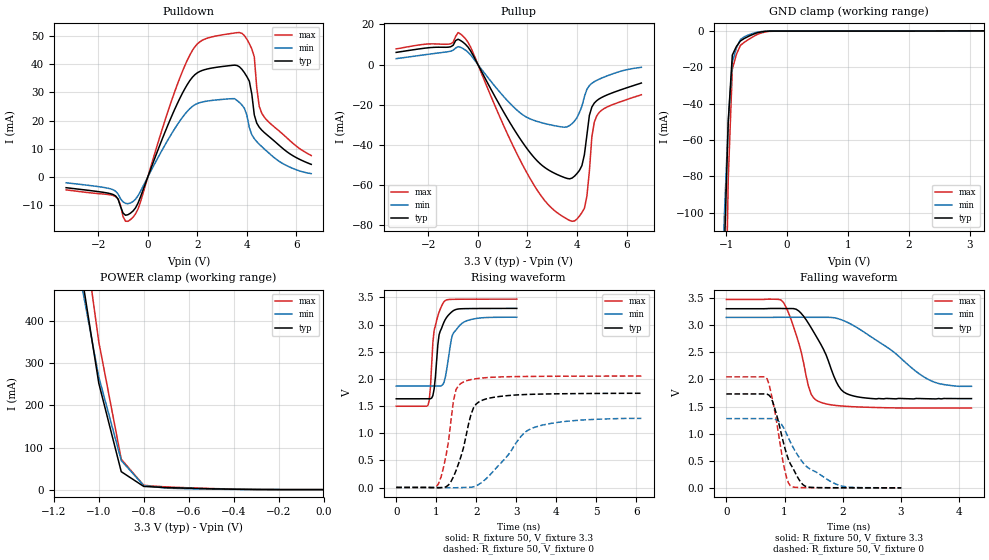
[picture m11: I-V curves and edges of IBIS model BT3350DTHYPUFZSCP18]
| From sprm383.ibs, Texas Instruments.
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|   Model Cell BT3350DTHYPUFZSCP18
[Model]   BT3350DTHYPUFZSCP18
Model_type   I/O
Polarity   Non-Inverting
Enable   Active-Low
Vinl =  0.8V
Vinh =  2V
Cref =  15.0000pF
Rref =  100.0000M
Vref =  0V
Vmeas =  1.65
C_comp   1.486782p   1.450653p   1.527115p
[Model Spec]
Vinl   0.8V   0.8V   0.8V
Vinh   2V   2V   2V
[Temperature Range]   25   105   0
[Voltage Range]   3.3   3.14   3.47
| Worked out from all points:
|   slope of the pulldown table from 0 to 0.495 V, typ, clamps not added: 43 ohm
|   slope of the pullup table from 0 to 0.495 V, typ, clamps not added: 42.8 ohm
|   GND clamp passes 1 mA (typ) near -0.48 V on its own axis
|   POWER clamp passes 1 mA (typ) near -0.41 V on its own axis
|   rising waveform, R_fixture 50, V_fixture 3.3: 20-80 % time 180ps typ, 223ps min, 150ps max; typ from 1.64 V to 3.3 V
|   rising waveform, R_fixture 50, V_fixture 0: 20-80 % time 378ps typ, 854ps min, 250ps max; typ from 0.003 V to 1.74 V
|   falling waveform, R_fixture 50, V_fixture 3.3: 20-80 % time 434ps typ, 942ps min, 290ps max; typ from 3.3 V to 1.65 V
|   falling waveform, R_fixture 50, V_fixture 0: 20-80 % time 298ps typ, 570ps min, 197ps max; typ from 1.73 V to 0.004 V
[POWER_clamp]
|   voltage   I(typ)   I(min)   I(max)
-3.3V     9.961A     8.611A     10.94A
-1.067V   478.9mA    459.3mA    610.8mA
-1.033V   365.9mA    363.6mA    481.1mA
-1V       253mA      268mA      351.4mA
-900mV    42.61mA    69.09mA    72.29mA
-800mV    7.588mA    9.637mA    10.15mA
-700mV    4.837mA    3.413mA    6.304mA
-600mV    3.264mA    2.054mA    4.281mA
-300mV    294.4uA    124uA      421.6uA
-11.55fV  111.8nA    122.7nA    532.3nA
[Pulldown]
|   voltage   I(typ)   I(min)   I(max)
-3.3V     -3.799mA   -2.054mA   -4.568mA
-1.3V     -6.728mA   -5.045mA   -6.952mA
-700mV    -12.84mA   -9.218mA   -15.12mA
-400mV    -9.372mA   -6.707mA   -11.45mA
900mV     20.28mA    14.47mA    25.55mA
1.8V      35.39mA    25.05mA    44.9mA
3.6V      39.59mA    27.18mA    51.23mA
4.1V      33.99mA    17.52mA    47.31mA
4.3V      22.03mA    13.6mA     42.63mA
4.4V      19.11mA    12.56mA    31.7mA
4.6V      16.65mA    10.8mA     22.67mA
6.6V      4.483mA    1.197mA    7.628mA
[Pullup]
|   voltage   I(typ)   I(min)   I(max)
-3.3V     6.066mA    2.957mA    7.802mA
-600mV    11.14mA    7.958mA    14.14mA
1.3V      -29.12mA   -19.42mA   -37.44mA
2.2V      -45.34mA   -27.53mA   -58.77mA
2.9V      -52.9mA    -29.98mA   -70.61mA
3.8V      -56.58mA   -29.42mA   -78.12mA
4.3V      -44.86mA   -15.96mA   -71.64mA
4.4V      -35.19mA   -12.35mA   -65.67mA
4.5V      -25.37mA   -10.47mA   -53.29mA
4.6V      -21.19mA   -9.34mA    -36.14mA
4.8V      -17.96mA   -7.847mA   -25.51mA
6.6V      -9.2mA     -1.379mA   -15.05mA
[GND_clamp]
|   voltage   I(typ)   I(min)   I(max)
-3.3V     -13.48A    -11.6A     -14.64A
-1.1V     -237.6mA   -179.7mA   -391.1mA
-1.033V   -124.3mA   -104mA     -204.7mA
-966.7mV  -49.58mA   -49.82mA   -81.35mA
-900mV    -13.35mA   -17.24mA   -21.09mA
-833.3mV  -8.63mA    -9.469mA   -12.94mA
-766.7mV  -5.563mA   -4.788mA   -7.981mA
-700mV    -4.145mA   -3.193mA   -6.208mA
-500mV    -1.148mA   -798uA     -2.146mA
-300mV    -166.1uA   -102.4uA   -290.3uA
3.233V    -8.734uA   9.395uA    -38.37uA
[Ramp]
| variable   typ   min   max
dV/dt_f   1.026406/0.448073n   0.8129736/1.011668n   1.202557/0.2908703n
dV/dt_r   1.048978/0.378546n   0.79136/0.9065475n   1.235918/0.2476382n
R_load = 50
[Rising Waveform]
R_fixture = 50
V_fixture = 3.3
V_fixture_min = 3.14
V_fixture_max = 3.47
|   time   V(typ)   V(min)   V(max)
0s        1.635V     1.869V     1.498V
796ps     1.636V     1.87V      1.519V
856ps     1.636V     1.87V      1.854V
916ps     1.694V     1.87V      2.674V
948ps     1.818V     1.87V      2.898V
1.072ns   2.817V     1.87V      3.232V
1.224ns   3.092V     2.02V      3.443V
1.408ns   3.247V     2.815V     3.466V
1.624ns   3.293V     3.013V     3.468V
3.012ns   3.299V     3.137V     3.47V
[Rising Waveform]
R_fixture = 50
V_fixture = 0
V_fixture_min = 0
V_fixture_max = 0
|   time   V(typ)   V(min)   V(max)
0s        3.11mV     1.91mV     3.799mV
1.056ns   -4.79mV    1.888mV    70.22mV
1.244ns   13.87mV    330.7uV    588.2mV
1.432ns   202.3mV    -4.369mV   1.607V
1.496ns   316mV      -2.82mV    1.805V
1.684ns   743mV      1.97mV     1.946V
1.932ns   1.47V      13.69mV    1.997V
2.244ns   1.632V     162mV      2.024V
3.432ns   1.718V     1.103V     2.047V
6.124ns   1.736V     1.275V     2.053V
[Falling Waveform]
R_fixture = 50
V_fixture = 3.3
V_fixture_min = 3.14
V_fixture_max = 3.47
|   time   V(typ)   V(min)   V(max)
0s        3.3V       3.14V      3.47V
984ps     3.303V     3.143V     3.411V
1.244ns   3.259V     3.143V     2.669V
1.412ns   3.029V     3.142V     1.87V
1.456ns   2.952V     3.142V     1.73V
1.584ns   2.72V      3.141V     1.594V
1.928ns   1.878V     3.114V     1.515V
2.1ns     1.723V     3.039V     1.502V
3.476ns   1.643V     1.996V     1.472V
4.212ns   1.647V     1.872V     1.473V
[Falling Waveform]
R_fixture = 50
V_fixture = 0
V_fixture_min = 0
V_fixture_max = 0
|   time   V(typ)   V(min)   V(max)
0s        1.732V     1.278V     2.046V
700ps     1.729V     1.278V     2.01V
792ps     1.6V       1.277V     1.629V
916ps     1.128V     1.214V     869.4mV
1.008ns   727.3mV    1.06V      307.7mV
1.1ns     445.6mV    847.2mV    42.67mV
1.252ns   150.8mV    561.8mV    10.05mV
1.344ns   41.15mV    433.4mV    7.839mV
1.896ns   6.131mV    68.56mV    4.859mV
3.004ns   4.329mV    5.06mV     4.055mV
